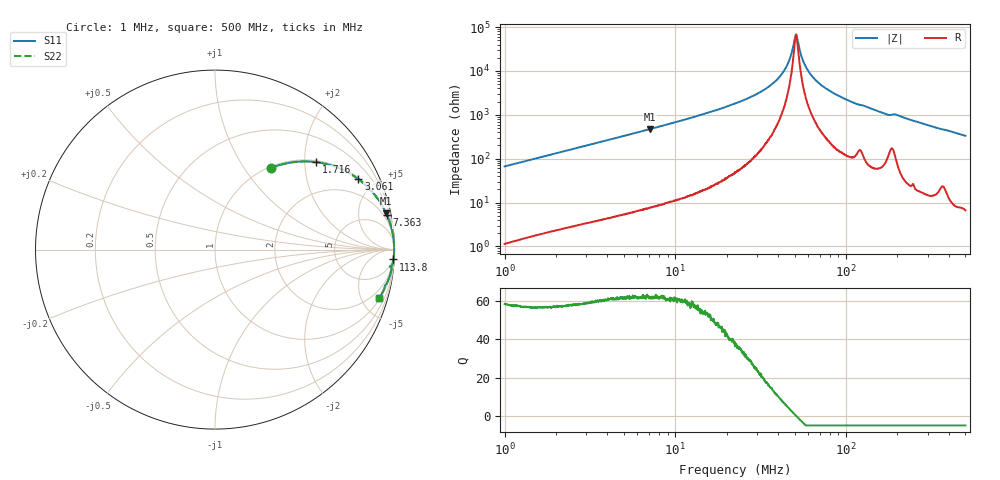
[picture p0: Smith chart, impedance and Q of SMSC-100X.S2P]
!s-Parameter Generated by FASTRON Sdn. Bhd.
!FASTRON P/N : SMSC-100X
!Keysight Technologies,E4991B,MY54100416,A.01.15
!Date: Mon Mar 16 10:17:34 2026
!Version  : Rev00 Mon Mar 16 10:17:34 2026
!Data & Calibration Information:
!PortZ  Port1:50+j0  Port2:50+j0
!When reading, reference impedance value at option line is always used.
!Remarks : This data is being provided solely for informational purposes.
!Freq	S11	S21	S12	S22
# Hz S dB R 50
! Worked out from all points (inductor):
!   1601 points, 1 MHz to 500 MHz, reference 50 ohm
!   read as one part in series: L = 10.6 uH near 1.032 MHz
!   highest Q = 62.3 at 7.082 MHz (marker M1), where L = 10.6 uH
!   self-resonance near 50.94 MHz
!   S11 on the Smith chart (normalised r, x): 1 MHz: 1.02, +1.33; 1.716 MHz: 1.04, +2.28; 3.061 MHz: 1.07, +4.04; 7.363 MHz: 1.16, +9.82; 113.8 MHz: 3, -36; 500 MHz: 1.13, -6.66
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1000000  -5.18 55.6  -1.67 -33.4  -1.67 -33.4  -5.18 55.6
1715825  -2.56 40.9  -3.68 -48.1  -3.68 -48.1  -2.56 40.9
2820919  -1.16 28.0  -6.57 -61.0  -6.57 -61.0  -1.16 28.0
3060657  -1.01 26.1  -7.12 -62.9  -7.12 -62.9  -1.01 26.1
7082320  -0.22 11.9  -13.70 -77.2  -13.70 -77.2  -0.22 11.9
7362819  -0.20 11.5  -14.03 -77.6  -14.03 -77.6  -0.20 11.5
7957584  -0.18 10.6  -14.70 -78.5  -14.70 -78.5  -0.18 10.6
2.236068e7  -0.03 3.2  -25.13 -85.2  -25.13 -85.2  -0.03 3.2
3.171773e7  -0.02 1.7  -30.55 -85.5  -30.55 -85.5  -0.02 1.7
3.988656e7  -0.01 0.9  -36.48 -83.6  -36.48 -83.6  -0.01 0.9
4.551764e7  -0.01 0.4  -43.15 -77.3  -43.15 -77.3  -0.01 0.4
4.977112e7  -0.01 0.1  -53.86 -43.8  -53.86 -43.8  -0.01 0.1
5.074715e7  -0.01 0.0  -56.41 -8.7  -56.41 -8.7  -0.01 0.0
5.194369e7  -0.01 -0.1  -54.34 36.2  -54.34 36.2  -0.01 -0.1
5.484648e7  -0.01 -0.3  -46.57 70.6  -46.57 70.6  -0.01 -0.3
5.679767e7  -0.01 -0.4  -43.45 76.1  -43.45 76.1  -0.01 -0.4
6.307767e7  -0.01 -0.7  -37.72 82.0  -37.72 82.0  -0.01 -0.7
7.870937e7  -0.02 -1.6  -31.33 84.4  -31.33 84.4  -0.02 -1.6
1.138355e8  -0.04 -3.2  -25.16 83.1  -25.16 83.1  -0.04 -3.2
1.77937e8  -0.15 -5.7  -20.06 77.1  -20.06 77.1  -0.15 -5.7
1.953218e8  -0.13 -5.5  -20.25 78.7  -20.25 78.7  -0.13 -5.5
5e8  -0.42 -16.6  -10.87 72.2  -10.87 72.2  -0.42 -16.6
